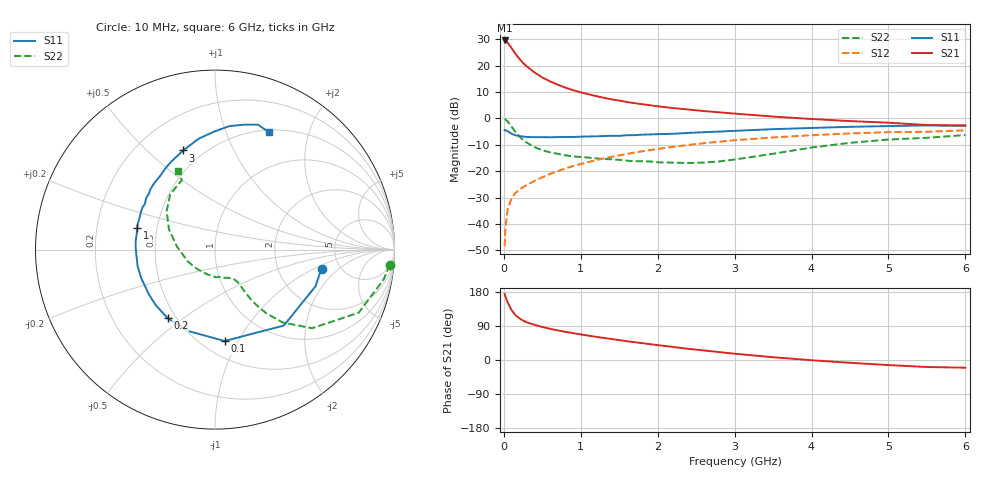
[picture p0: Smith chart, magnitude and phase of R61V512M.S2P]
! SIEMENS Small Signal Semiconductors
! BFR193
! Si NPN RF Bipolar Junction Transistor in SOT23
! VCE = 1.5 V  IC = 12 mA
! Common Emitter S-Parameters:  May  1996
# GHz  S  MA  R  50
!  f  S11  S21  S12  S22
! GHz  MAG  ANG  MAG  ANG  MAG  ANG  MAG  ANG
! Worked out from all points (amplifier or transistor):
!   36 points, 10 MHz to 6 GHz, reference 50 ohm
!   highest |S21| = 29.5 dB at 10 MHz (marker M1)
!   |S21| within 3 dB of that: start of sweep to 102.7 MHz
!   unconditionally stable (mu >= 1): 659.9 MHz to 2.049 GHz
!   at 250 MHz: K = 0.71, MSG = 23.5 dB, |S12| = -26.0 dB
!   at 1.4 GHz: K = 1.04, MAG = 9.7 dB, |S12| = -14.6 dB
!   at 6 GHz: K = 0.96, MSG = 0.9 dB, |S12| = -4.5 dB
!   S11 on the Smith chart (normalised r, x): 10 MHz: 3.61, -1.20; 100 MHz: 0.64, -0.88; 200 MHz: 0.45, -0.44; 1 GHz: 0.38, +0.12; 3 GHz: 0.39, +0.65; 6 GHz: 0.52, +1.42
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0.01  0.6027 -10.1  29.9 174.1  0.0038 86.4  0.9769 -5.0
0.02  0.596 -20.1  29.83 167.7  0.0081 82.8  0.9541 -10.1
0.05  0.5711 -47.8  27.29 151.6  0.0188 71.5  0.8746 -23.7
0.1  0.5122 -84.0  21.44 131.9  0.0309 60.7  0.6959 -39.0
0.15  0.4776 -108.7  16.83 118.4  0.0387 57.0  0.5528 -47.2
0.2  0.4637 -124.8  13.58 110.2  0.0439 56.2  0.4564 -51.1
0.25  0.4526 -137.1  11.23 104.0  0.0499 56.4  0.3915 -53.1
0.3  0.4444 -146.2  9.589 99.3  0.055 57.6  0.3455 -54.2
0.4  0.4407 -159.0  7.39 92.7  0.0655 59.9  0.2847 -54.8
0.5  0.441 -168.0  5.959 87.1  0.0766 61.7  0.2488 -54.7
0.6  0.4388 -175.3  5.03 82.3  0.0886 62.6  0.2277 -54.9
0.7  0.4422 178.5  4.355 78.0  0.1001 63.3  0.2128 -55.7
0.8  0.4445 173.9  3.828 74.4  0.1122 63.4  0.1997 -56.9
1  0.4505 164.3  3.11 67.5  0.1365 63.3  0.1853 -59.4
1.1  0.4544 160.8  2.858 64.3  0.1493 62.9  0.1808 -62.0
1.6  0.4797 143.1  2.037 49.5  0.2125 58.7  0.1584 -77.5
2.2  0.5113 126.8  1.567 34.4  0.289 51.7  0.145 -105.6
3  0.5801 107.8  1.231 16.6  0.3855 40.1  0.1661 -157.3
3.5  0.625 98.3  1.083 7.3  0.4353 32.3  0.2138 175.0
4.5  0.692 83.5  0.889 -7.4  0.5191 17.7  0.3444 141.4
5.5  0.7359 71.1  0.749 -18.5  0.5582 2.8  0.4289 115.5
6  0.7206 65.5  0.735 -20.3  0.5935 -1.5  0.4829 115.6
